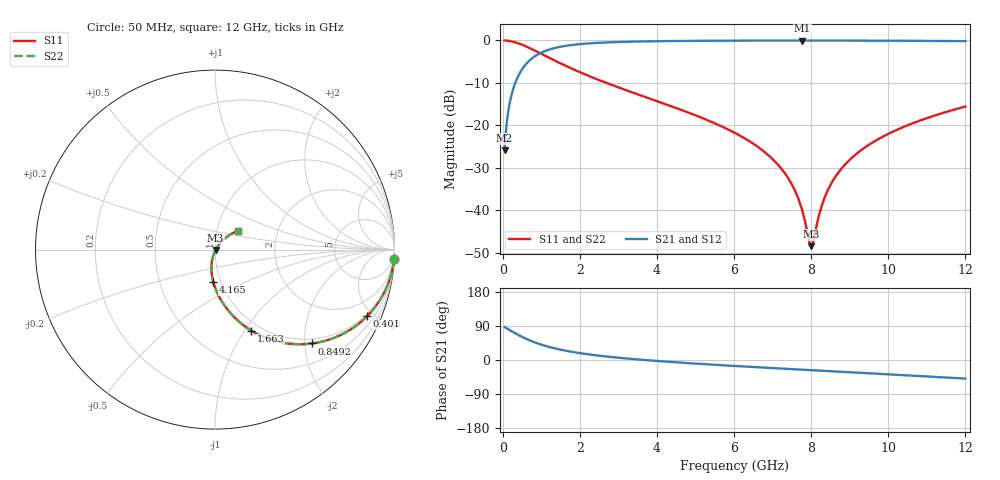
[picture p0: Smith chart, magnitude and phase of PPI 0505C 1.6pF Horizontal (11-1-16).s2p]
# MHz S MA R 50
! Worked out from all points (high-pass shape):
!   1601 points, 50 MHz to 12 GHz, reference 50 ohm
!   highest |S21| = -0.04 dB at 7.773 GHz (marker M1); lowest = -25.9 dB at 50 MHz (marker M2)
!   |S21| within 3 dB of the highest: 966.6 MHz to end of sweep
!   lowest |S11| = -48.5 dB at 8.004 GHz (marker M3), VSWR 1.01, Z = 50.3 - j0.17 ohm
!   |S11| at or under -10 dB: 2.686 GHz to end of sweep
!   |S22| runs from -48.5 to 0.0 dB; largest |S21 - S12| = 0
!   S11 on the Smith chart (normalised r, x): 50 MHz: 1, -37; 401 MHz: 0.90, -4.61; 849.2 MHz: 0.90, -2.16; 1.663 GHz: 0.90, -1.08; 4.165 GHz: 0.92, -0.34; 12 GHz: 1.26, +0.27
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50  0.9987 -3.1  0.0509 86.9  0.0509 86.9  0.9987 -3.1
199.375  0.9799 -12.2  0.1992 77.8  0.1992 77.8  0.9799 -12.2
401.0312  0.9252 -23.6  0.3789 66.3  0.3789 66.3  0.9252 -23.6
849.1562  0.7528 -44.0  0.657 45.9  0.657 45.9  0.7528 -44.0
1237.531  0.6137 -56.2  0.7879 33.6  0.7879 33.6  0.6137 -56.2
1663.25  0.4951 -65.8  0.8669 24.0  0.8669 24.0  0.4951 -65.8
2044.156  0.4146 -72.2  0.9079 17.5  0.9079 17.5  0.4146 -72.2
4038.312  0.1898 -92.0  0.9789 -2.8  0.9789 -2.8  0.1898 -92.0
4165.281  0.181 -92.9  0.9805 -3.8  0.9805 -3.8  0.181 -92.9
6025  0.08119 -103.5  0.9931 -15.8  0.9931 -15.8  0.08119 -103.5
6682.25  0.05297 -105.9  0.9948 -19.5  0.9948 -19.5  0.05297 -105.9
7175.188  0.03293 -106.2  0.9955 -22.3  0.9955 -22.3  0.03293 -106.2
7526.219  0.0191 -103.3  0.9957 -24.3  0.9957 -24.3  0.0191 -103.3
7772.688  0.009775 -93.4  0.9958 -25.6  0.9958 -25.6  0.009775 -93.4
7944.469  0.004407 -58.3  0.9957 -26.6  0.9957 -26.6  0.004407 -58.3
8004.219  0.003768 -26.6  0.9957 -26.9  0.9957 -26.9  0.003768 -26.6
8019.156  0.00382 -17.8  0.9957 -27.0  0.9957 -27.0  0.00382 -17.8
8325.375  0.01315 44.3  0.9955 -28.6  0.9955 -28.6  0.01315 44.3
8661.469  0.026 50.7  0.9952 -30.5  0.9952 -30.5  0.026 50.7
9214.156  0.04764 51.5  0.9942 -33.5  0.9942 -33.5  0.04764 51.5
10013.31  0.07978 49.0  0.9918 -37.9  0.9918 -37.9  0.07978 49.0
12000  0.1665 39.2  0.9802 -49.0  0.9802 -49.0  0.1665 39.2
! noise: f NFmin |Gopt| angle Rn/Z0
50  0.0009255  0.956  1.718  0.004739
1372  0.005214  0.7435  6.498  0.004066
2701  0.00808  0.684  10.64  0.004916
4031  0.01059  0.6488  14.81  0.005635
5360  0.01295  0.6255  18.93  0.006306
6682  0.01523  0.61  22.96  0.006971
8012  0.01753  0.6001  26.91  0.007666
9341  0.01987  0.5949  30.76  0.008415
1.067e+04  0.02231  0.5935  34.49  0.009243
1.2e+04  0.02488  0.5957  38.12  0.01018
